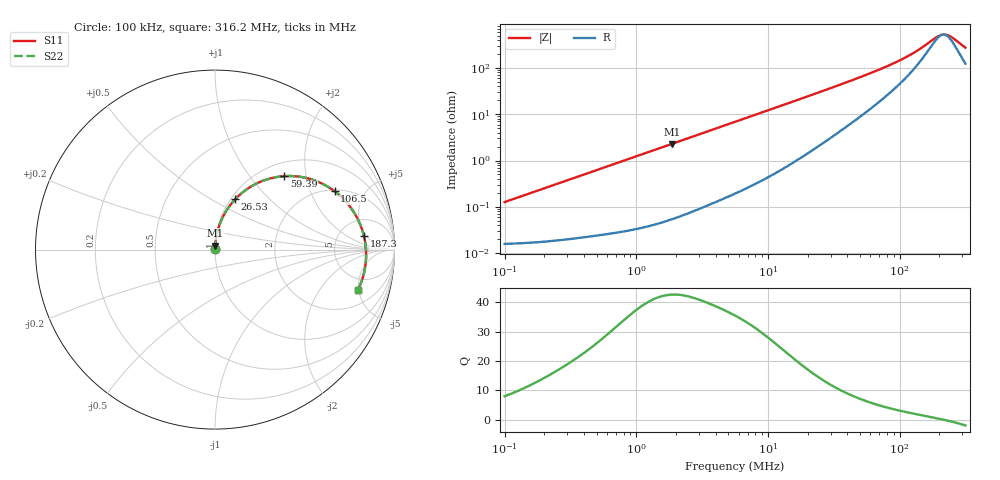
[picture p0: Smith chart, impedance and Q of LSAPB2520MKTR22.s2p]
! LSAPB2520MKTR22  S-PARAMETER MODEL  ( General Type )
! Model Generated by TAIYO YUDEN Corporation (http://www.ty-top.com)
! Version 2.0
! TAIYO YUDEN Control No. 20210629
! Copyright(c) 2015 TAIYO YUDEN CO.,LTD. All Rights Reserved.
! Product Description (link to TY-COMPAS)
! https://ds.yuden.co.jp/TYCOMPAS/or/detail?pn=LSAPB2520MKTR22M&u=M
! Products Name : Inductors
! Characteristics :
!  Inductance : 0.22 uH , SRF(min) : -Hz , DC Resistance(max) : 0.021 Ohm
!  Rated Current : Saturation :7500 mA , Temp Rise : 5000 mA (40 degC)
!  Case Size : 2.5 x 2.0 / 0.098 x 0.079 [mm/inch] , Thickness : 1.2 / 0.047 [mm/inch]
!  (Conditions: Temperature = 25 degC , DC Bias Current/Voltage = 0A / 0V)
! External Node Assignments :
!  1  o---GGG---o  2
! GND o---------o GND
! Frequency Range : 0.1MHz  -  316.199832MHz  [ 402 STEP ]
# MHz S RI R 50
! Freq[MHz].  S11 Real  S11 Imag  S21 Real  S21 Imag  S12 Real  S12 Imag  S22 Real  S22 Imag
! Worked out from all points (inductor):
!   401 points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, 100 kHz to 316.2 MHz, reference 50 ohm
!   read as one part in series: L = 200 nH near 104.1 kHz
!   highest Q = 42.6 at 1.857 MHz (marker M1), where L = 195 nH
!   self-resonance near 214.6 MHz
!   S11 on the Smith chart (normalised r, x): 100 kHz: 1.00, +0.00; 26.53 MHz: 1.05, +0.65; 59.39 MHz: 1.26, +1.50; 106.5 MHz: 2.07, +3.00; 187.3 MHz: 8.84, +4.34; 316.2 MHz: 3.48, -4.91
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0.1  0.000159 0.00126  0.9998 -0.00126  0.9998 -0.00126  0.000159 0.00126
0.385695  0.000239 0.00479  0.9998 -0.00479  0.9998 -0.00479  0.000239 0.00479
1.487603  0.000771 0.0183  0.9992 -0.0183  0.9992 -0.0183  0.000771 0.0183
1.856676  0.00105 0.0227  0.9989 -0.0227  0.9989 -0.0227  0.00105 0.0227
5.623165  0.00654 0.0677  0.9935 -0.0677  0.9935 -0.0677  0.00654 0.0677
11.38223  0.0236 0.1338  0.9764 -0.1338  0.9764 -0.1338  0.0236 0.1338
16.03156  0.0447 0.1837  0.9553 -0.1837  0.9553 -0.1837  0.0447 0.1837
21.68824  0.0781 0.2388  0.9219 -0.2388  0.9219 -0.2388  0.0781 0.2388
26.52916  0.112 0.28  0.888 -0.28  0.888 -0.28  0.112 0.28
39.69369  0.2195 0.3621  0.7805 -0.3621  0.7805 -0.3621  0.2195 0.3621
59.39086  0.3861 0.4092  0.6139 -0.4092  0.6139 -0.4092  0.3861 0.4092
71.19815  0.4746 0.4056  0.5254 -0.4056  0.5254 -0.4056  0.4746 0.4056
83.65039  0.5544 0.3855  0.4456 -0.3855  0.4456 -0.3855  0.5544 0.3855
106.5287  0.6662 0.3253  0.3338 -0.3253  0.3338 -0.3253  0.6662 0.3253
138.4253  0.7631 0.2245  0.2369 -0.2245  0.2369 -0.2245  0.7631 0.2245
187.2682  0.8297 0.075  0.1703 -0.075  0.1703 -0.075  0.8297 0.075
207.116  0.8393 0.0198  0.1607 -0.0198  0.1607 -0.0198  0.8393 0.0198
220.0206  0.8418 -0.0142  0.1582 0.0142  0.1582 0.0142  0.8418 -0.0142
229.0673  0.8419 -0.0372  0.1581 0.0372  0.1581 0.0372  0.8419 -0.0372
248.292  0.8386 -0.0837  0.1614 0.0837  0.1614 0.0837  0.8386 -0.0837
303.7119  0.8074 -0.1998  0.1926 0.1998  0.1926 0.1998  0.8074 -0.1998
316.1998  0.7971 -0.2223  0.2029 0.2223  0.2029 0.2223  0.7971 -0.2223
